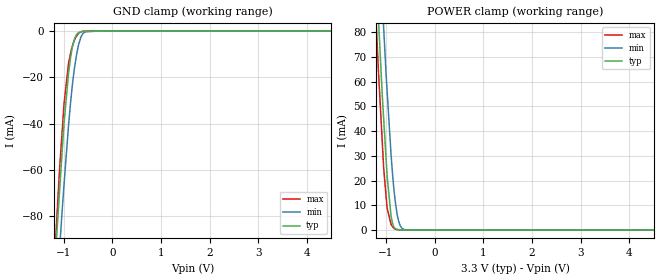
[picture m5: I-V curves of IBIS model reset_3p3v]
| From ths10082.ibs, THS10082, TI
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|   reset_3p3v Model
[Model]   reset_3p3v
Model_type   Input
Vinl = 0.6
Vinh = 2
|   typ   min   max
C_comp   1.027e-12   1.022e-12   1.043e-12
[Voltage Range]   3.3   3   3.6
|Ambient Temperature   25   85   -40
|Junction Temperature
[Temperature Range]   27   125   -40
[Power Clamp Reference]   3.3   3   3.6
[GND Clamp Reference]   0   0   0
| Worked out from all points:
|   GND clamp passes 1 mA (typ) near -0.71 V on its own axis
|   POWER clamp passes 1 mA (typ) near -0.83 V on its own axis
[GND Clamp]
|   Voltage   I(typ)   I(min)   I(max)
-3.3V     -973.3mA   -932.3mA   -1.035A
-1.162V   -95.19mA   -120.2mA   -89.81mA
-1.084V   -69.76mA   -95.18mA   -60.34mA
-1.035V   -53.91mA   -79.62mA   -45.29mA
-990mV    -39.87mA   -66.2mA    -31.36mA
-896.4mV  -17.98mA   -40.53mA   -13.69mA
-821.7mV  -7.21mA    -23.92mA   -6.726mA
-785.4mV  -4.002mA   -17.57mA   -4.472mA
-693mV    -706.4uA   -6.107mA   -935.9uA
-591mV    -125.6uA   -821.1uA   -75.2uA
-285mV    -60.21uA   -318.9nA   -93.3nA
6.6V      0A         0A         0A
[POWER Clamp]
|   Voltage   I(typ)   I(min)   I(max)
-3.3V     1.042A     1.058A     1.043A
-1.241V   118.6mA    156.6mA    99.74mA
-1.156V   85.07mA    122.2mA    64.04mA
-1.131V   75.39mA    112.3mA    55.04mA
-1.048V   44.55mA    81.16mA    24.76mA
-979.2mV  22.2mA     56.56mA    8.863mA
-897.6mV  5.699mA    30.6mA     2.3mA
-810mV    519.6uA    11.42mA    237.9uA
-768mV    211.5uA    5.922mA    135.6uA
-711mV    52.18uA    1.815mA    88.81uA
-591mV    9.743uA    71.96uA    15.49uA
6.6V      0A         0A         0A
